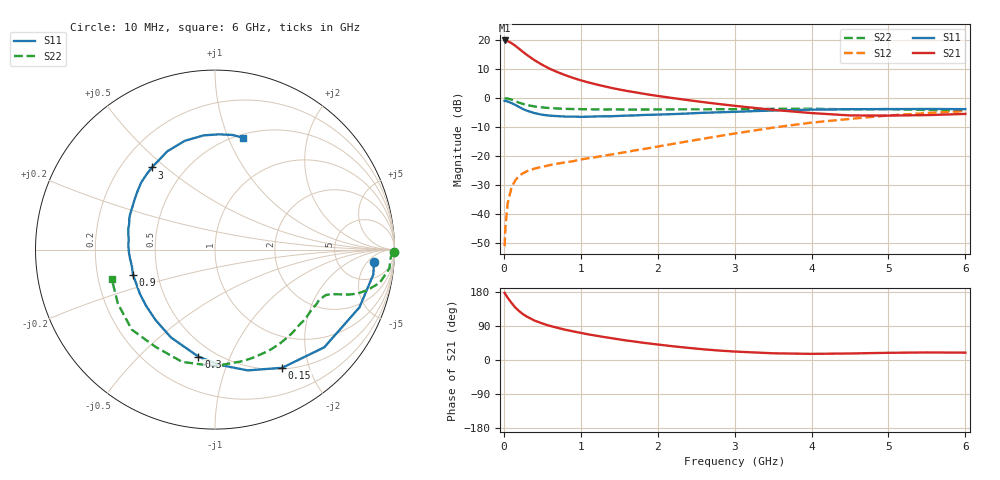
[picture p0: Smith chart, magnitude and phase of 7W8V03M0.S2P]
! Infineon Technologies  Discrete & RF Semiconductors
! BFS17W
! Si NPN RF Bipolar Junction Transistor in SOT323
! VCE = 8 V  IC = 3 mA
! Common Emitter S-Parameters:  August  1999
# GHz  S  MA  R  50
!  f  S11  S21  S12  S22
! GHz  MAG  ANG  MAG  ANG  MAG  ANG  MAG  ANG
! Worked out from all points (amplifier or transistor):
!   36 points, 10 MHz to 6 GHz, reference 50 ohm
!   highest |S21| = 19.8 dB at 10 MHz (marker M1)
!   |S21| within 3 dB of that: start of sweep to 205.3 MHz
!   unconditionally stable (mu >= 1): 740.6 MHz to 2.536 GHz; 4.944 GHz to end of sweep
!   at 250 MHz: K = 0.44, MSG = 20.9 dB, |S12| = -26.0 dB
!   at 1.4 GHz: K = 1.24, MAG = 8.5 dB, |S12| = -19.5 dB
!   at 6 GHz: K = 1.07, MAG = -2.1 dB, |S12| = -4.5 dB
!   S11 on the Smith chart (normalised r, x): 10 MHz: 12, -8; 150 MHz: 0.52, -1.60; 300 MHz: 0.41, -0.77; 900 MHz: 0.36, -0.13; 3 GHz: 0.33, +0.45; 6 GHz: 0.54, +1.14
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0.01  0.8888 -4.4  9.777 177.3  0.0028 84.8  0.9987 -0.8
0.02  0.8928 -9.0  9.72 173.7  0.0058 84.6  0.9798 -2.5
0.05  0.8667 -21.8  9.515 164.3  0.0155 78.0  0.9774 -6.2
0.1  0.8167 -41.8  8.787 150.6  0.0289 68.5  0.9358 -11.4
0.15  0.7574 -60.4  7.907 138.3  0.0383 60.3  0.8788 -14.9
0.2  0.697 -74.9  7.013 128.7  0.0459 56.2  0.8299 -17.2
0.25  0.6428 -87.7  6.19 120.8  0.0504 51.3  0.7884 -18.5
0.3  0.6035 -98.8  5.509 114.4  0.0548 49.2  0.7572 -19.3
0.4  0.5477 -116.6  4.458 104.0  0.0607 46.8  0.7122 -20.4
0.5  0.5137 -130.1  3.717 96.4  0.0651 46.3  0.6867 -21.3
0.6  0.4955 -140.8  3.168 90.0  0.0698 47.2  0.6689 -22.2
0.7  0.486 -149.3  2.774 84.7  0.0741 48.5  0.6585 -23.5
0.9  0.4779 -163.0  2.212 75.6  0.0813 51.7  0.6434 -26.5
1.1  0.4761 -174.0  1.851 67.5  0.0916 54.9  0.6375 -30.1
1.3  0.4835 177.0  1.595 60.7  0.1016 58.1  0.633 -34.1
1.6  0.4972 166.2  1.32 51.3  0.1175 62.2  0.6304 -40.5
2.2  0.527 148.4  0.994 36.2  0.1619 68.6  0.6357 -55.0
3  0.5772 127.5  0.732 22.3  0.2439 70.1  0.6404 -75.9
3.5  0.6086 115.9  0.624 17.7  0.3088 67.5  0.6493 -90.3
4.5  0.6396 95.7  0.5 17.2  0.4355 55.9  0.6353 -121.6
5.5  0.6462 81.2  0.506 19.9  0.5485 42.5  0.6193 -150.9
6  0.6419 75.7  0.531 19.4  0.5926 35.9  0.598 -164.1
